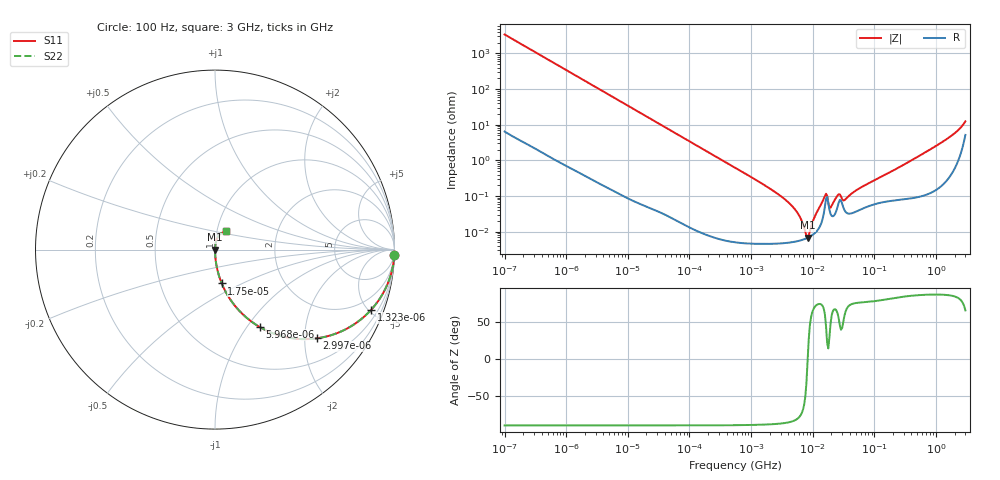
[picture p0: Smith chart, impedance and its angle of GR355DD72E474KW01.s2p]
!Murata Part Number: GR355DD72E474KW01
!These Parameters are Measured in Series Mode Connection
!Data Generated on Jun 19, 2026
!  o--ll--o
!Port1  Port2
!  o------o
!Operation Temp=25[degC], DC Bias Voltage=0[V]
!Freq. Start=100[Hz] Stop=3[GHz] 401[Steps]
# Hz S RI R 50
!Freq.(Hz) S11(Real) S11(Imag) S21(Real) S21(Imag) S12(Real) S12(Imag) S22(Real) S22(Imag)
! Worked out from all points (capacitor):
!   401 points, 100 Hz to 3 GHz, reference 50 ohm
!   read as one part in series: C = 466 nF near 109 Hz
!   lowest |Z| = 6.73 mohm at 8.245 MHz (marker M1)
!   series resonance near 8.282 MHz, so ESL is about 790 pH
!   S11 on the Smith chart (normalised r, x): 100 Hz: 1, -68; 1.323 kHz: 1.01, -5.18; 2.997 kHz: 1.01, -2.29; 5.968 kHz: 1.00, -1.15; 17.5 kHz: 1.00, -0.39; 3 GHz: 1.10, +0.23
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100  0.9991 -0.0293  0.000913 0.0293  0.000913 0.0293  0.9991 -0.0293
414  0.9853 -0.1192  0.0147 0.1192  0.0147 0.1192  0.9853 -0.1192
1323  0.8696 -0.3357  0.1304 0.3357  0.1304 0.3357  0.8696 -0.3357
1788  0.7854 -0.4095  0.2146 0.4095  0.2146 0.4095  0.7854 -0.4095
2997  0.5666 -0.4944  0.4334 0.4944  0.4334 0.4944  0.5666 -0.4944
5968  0.249 -0.4313  0.751 0.4313  0.751 0.4313  0.249 -0.4313
17504  0.0376 -0.1889  0.9624 0.1889  0.9624 0.1889  0.0376 -0.1889
31977  0.0118 -0.1063  0.9882 0.1063  0.9882 0.1063  0.0118 -0.1063
547723  8.97e-05 -0.00628  0.9999 0.00628  0.9999 0.00628  8.97e-05 -0.00628
3799590  4.89e-05 -0.000725  1 0.000725  1 0.000725  4.89e-05 -0.000725
5597215  5.4e-05 -0.000343  0.9999 0.000343  0.9999 0.000343  5.4e-05 -0.000343
7565221  6.3e-05 -7.91e-05  0.9999 7.91e-05  0.9999 7.91e-05  6.3e-05 -7.91e-05
8245314  6.72e-05 -3.9e-06  0.9999 3.9e-06  0.9999 3.9e-06  6.72e-05 -3.9e-06
9794414  7.96e-05 0.000153  0.9999 -0.000153  0.9999 -0.000153  7.96e-05 0.000153
1.572531e7  0.000498 0.000874  0.9995 -0.000874  0.9995 -0.000874  0.000498 0.000874
2.035898e7  0.000276 0.000464  0.9997 -0.000464  0.9997 -0.000464  0.000276 0.000464
2.52476e7  0.000495 0.000912  0.9995 -0.000912  0.9995 -0.000912  0.000495 0.000912
3.412477e7  0.000359 0.000732  0.9996 -0.000732  0.9996 -0.000732  0.000359 0.000732
5.719833e7  0.000406 0.00159  0.9996 -0.00159  0.9996 -0.00159  0.000406 0.00159
1.751444e8  0.000739 0.00449  0.9993 -0.00449  0.9993 -0.00449  0.000739 0.00449
1.324213e9  0.00334 0.0343  0.9967 -0.0343  0.9967 -0.0343  0.00334 0.0343
3e9  0.0602 0.1011  0.9398 -0.1011  0.9398 -0.1011  0.0602 0.1011
